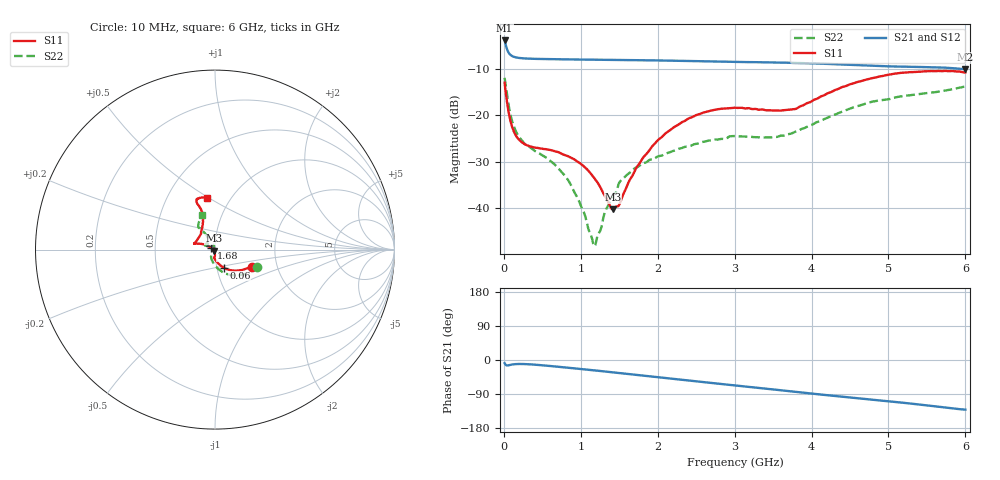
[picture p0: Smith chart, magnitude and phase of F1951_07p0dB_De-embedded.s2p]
! Integrated Device Technology
! Corporate Headquarters
! 6024 Silver Creek Valley Road
! San Jose, CA 95138  USA
! Phone:  1-408-284-8200
! Toll Free:  1-800-223-1366
! Webpage:  http://www.idt.com/
! Timing and RF Division
! 515 Groton Road, Suite 102
! Westford, MA 01886-6024
! Device:  F1951
! Description: 6-bit 0.5 dB Digital Step Attenuator
! Frequency:  100.0 -  4000.00 MHz
! Package:  4x4 mm Thin QFN Plastic Package: 24 pin
! Ports:  2 RF, 6 DC
!  Pin  1  = NC
!  Pin  2  = RF1  =  Port 1
!  Pin  3  = GND
!  Pin  4  = NC
!  Pin  5  = Serial Data Out (SDO)
!  Pin  6  = NC
!  Pin  7  = Reset Bar ( RSTb)
!  Pin  8  = Clock (CLK)
!  Pin  9  = Chip Select Bar (CSb)
!  Pin 10  = NC
!  Pin 11  = Serial Data In (SDI)
!  Pin 12  = NC
!  Pin 13  = NC
!  Pin 14  = VDD
!  Pin 15  = NC
!  Pin 16  = GND
!  Pin 17  = RF2  =  Port 2
!  Pin 18  = NC
!  Pin 19  = GND
!  Pin 20  = GND
!  Pin 21  = GND
!  Pin 22  = GND
!  Pin 23  = GND
!  Pin 24  = GND
! State:  14
! Atten State:  7.0 dB
! Voltage:  +3.30 Volts
! Current:  0.475 mA
! Data:  The device was measured on a F195X evaluation board which has
!  individual transmission lines to the RF pins.  Data was collected
!  de-embedded using a Automatic Fixture Removal [AFR] (Keysight Technologies).
!  The reference plane is the edge of the package pin.
! Misc:  Lot Code  1225BCA
!  Action Tracker AT0399
! Date Measured:  2018-09-13
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# GHz S dB R 50
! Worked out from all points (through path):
!   600 points, 10 MHz to 6 GHz, reference 50 ohm
!   highest |S21| = -3.85 dB at 10 MHz (marker M1); lowest = -10.0 dB at 6 GHz (marker M2)
!   group delay of S21, straight-line fit = 58.5 ps
!   lowest |S11| = -40.2 dB at 1.42 GHz (marker M3), VSWR 1.02, Z = 49.2 - j0.603 ohm
!   |S11| at or under -10 dB: start of sweep to end of sweep
!   |S22| runs from -48.2 to -11.9 dB; largest |S21 - S12| = 0.0006
!   S11 on the Smith chart (normalised r, x): 10 MHz: 1.48, -0.30; 60 MHz: 1.08, -0.22; 1.68 GHz: 0.96, +0.02; 6 GHz: 0.78, +0.49
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0.01  -12.92 -25.3  -3.85 -8.3  -3.84 -8.3  -11.89 -21.8
0.06  -19.09 -64.6  -6.42 -14.0  -6.42 -14.0  -17.64 -71.6
0.13  -23.48 -82.4  -7.37 -11.3  -7.37 -11.3  -22.36 -96.5
0.24  -25.86 -93.2  -7.69 -10.5  -7.69 -10.5  -25.54 -112.8
0.77  -28.42 -92.1  -7.91 -19.1  -7.91 -19.1  -32.56 -123.5
1.01  -30.58 -88.2  -7.97 -24.0  -7.97 -24.0  -39.85 -127.4
1.15  -32.96 -91.3  -7.98 -26.8  -7.98 -26.8  -46.79 -166.5
1.18  -33.63 -92.8  -7.99 -27.4  -7.99 -27.5  -48.20 169.1
1.25  -35.36 -97.9  -7.99 -28.9  -8.00 -28.9  -44.99 131.7
1.33  -37.82 -111.0  -8.00 -30.7  -8.01 -30.7  -40.25 114.3
1.42  -40.24 -141.0  -8.03 -32.6  -8.03 -32.6  -37.07 106.2
1.5  -39.26 -172.9  -8.05 -34.2  -8.05 -34.2  -34.51 108.6
1.68  -32.76 157.1  -8.07 -38.2  -8.07 -38.2  -31.69 108.1
2.01  -25.24 153.7  -8.16 -45.5  -8.16 -45.5  -28.80 122.1
2.49  -20.00 160.2  -8.30 -56.0  -8.30 -56.0  -26.17 145.4
3.01  -18.34 164.3  -8.47 -67.1  -8.48 -67.1  -24.44 155.5
3.55  -18.93 147.2  -8.60 -78.8  -8.60 -78.8  -24.64 137.3
3.79  -18.62 131.4  -8.71 -84.0  -8.71 -84.0  -23.52 127.3
4.01  -16.86 119.2  -8.79 -88.8  -8.79 -88.8  -22.00 121.5
4.5  -13.30 109.1  -9.11 -99.1  -9.11 -99.1  -18.56 122.8
5.01  -11.23 111.2  -9.43 -109.2  -9.44 -109.2  -16.50 126.6
6  -10.76 98.8  -10.05 -130.9  -10.05 -130.9  -13.76 110.9
